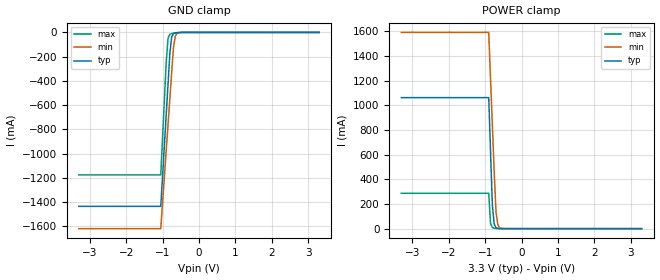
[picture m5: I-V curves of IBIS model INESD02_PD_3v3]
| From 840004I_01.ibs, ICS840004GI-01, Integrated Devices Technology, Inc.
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[Model] INESD02_PD_3v3
Model_type   Input
Polarity   Non-Inverting
Vinl = 0.80V
Vinh = 2.0V
|   typ   min   max
C_comp   2pF   1.5pF   2.5pF
|   typ   min   max
[Voltage range]  3.3V   3.15V   3.45V
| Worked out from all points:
|   GND clamp passes 1 mA (typ) near -0.56 V on its own axis
|   POWER clamp passes 1 mA (typ) near -0.61 V on its own axis
[GND_clamp]
|Voltage   I(typ)   I(min)   I(max)
-3.3V     -1.436A    -1.62A     -1.176A
-1.05V    -1.436A    -1.62A     -1.176A
-900mV    -678.5mA   -975.1mA   -244mA
-850mV    -426.1mA   -760.1mA   -46.85mA
-800mV    -173.9mA   -545.4mA   -16.11mA
-750mV    -36.96mA   -330.7mA   -9.916mA
-700mV    -9.696mA   -120.2mA   -7.056mA
-650mV    -3.545mA   -29.7mA    -4.857mA
-600mV    -1.629mA   -7.52mA    -3.049mA
-400mV    -52.81uA   -52.52uA   -108.7uA
3.3V      71.13uA    77.43uA    62.11uA
[POWER_clamp]
|Voltage   I(typ)   I(min)   I(max)
-3.3V     1.063A     1.593A     287.3mA
-900mV    1.063A     1.593A     287.3mA
-850mV    620.5mA    1.215A     41.84mA
-800mV    191.6mA    837.5mA    8.757mA
-750mV    37.76mA    460.2mA    3.328mA
-700mV    8.104mA    133.8mA    1.728mA
-650mV    2.076mA    32.66mA    905.3uA
-600mV    678.1uA    8.083mA    443.8uA
-450mV    104.2uA    213.3uA    89.09uA
3.3V      -3.041nA   -3.986uA   0A
